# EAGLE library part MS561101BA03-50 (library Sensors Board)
BAROMETRIC PRESSURE SENSOR
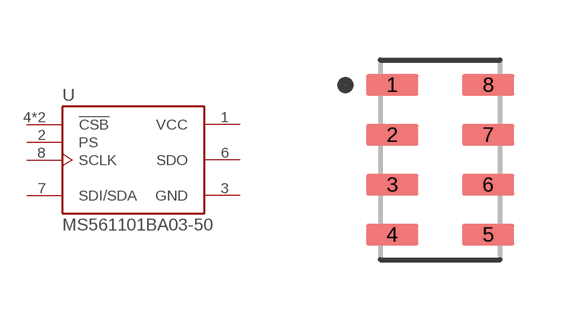
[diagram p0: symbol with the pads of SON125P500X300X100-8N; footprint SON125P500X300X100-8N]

Designator prefix U

## MS561101BA03-50 (AVAILABILITY: Unavailable; COMMENT: MS561101BA03-50; DESCRIPTION: Barometric Pressure Sensor; EU_ROHS_COMPLIANCE: Compliant; MF: TE Connectivity; MP: MS561101BA03-50; PACKAGE: SMD-8 TE Connectivity; PRICE: None; TE_PURCHASE_URL: https://www.te.com/usa-en/product-MS561101BA03-50.html?te_bu=Cor&te_type=disp&te_campaign=seda_glo_cor-seda-global-disp-prtnr-fy19-seda-model-bom-cta_sma-317_1&elqCampaignId=32493)  [SON125P500X300X100-8N]
1  VCC  pwr
2  PS  in
3  GND  pwr
4  !CSB  in
5  !CSB  in
6  SDO  out
7  SDI/SDA
8  SCLK  in

## Footprint SON125P500X300X100-8N (pad centres in mm)
smd 1.31 x 0.53: 1 -1.2,1.875; 2 -1.2,0.625; 3 -1.2,-0.625; 4 -1.2,-1.875; 5 1.2,-1.875; 6 1.2,-0.625; 7 1.2,0.625; 8 1.2,1.875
